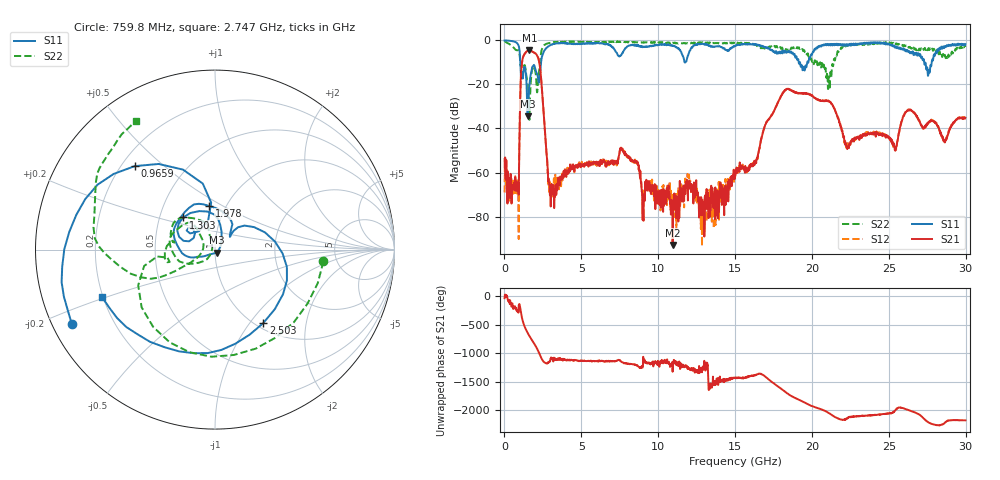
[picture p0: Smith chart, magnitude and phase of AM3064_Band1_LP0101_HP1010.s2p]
# Hz S DB R 50.0
!freq dBS11 angS11 dBS21 angS21 dBS12 angS12 dBS22 angS22
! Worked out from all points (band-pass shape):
!   1600 points, 10 MHz to 29.98 GHz, reference 50 ohm
!   highest |S21| = -4.58 dB at 1.622 GHz (marker M1); lowest = -92.9 dB at 10.94 GHz (marker M2)
!   |S21| within 3 dB of the highest: 1.212 GHz to 2.173 GHz (961.5 MHz wide, 56.8 % of centre)
!   lowest |S11| = -34.4 dB at 1.51 GHz (marker M3), VSWR 1.04, Z = 50.8 - j1.73 ohm
!   |S11| at or under -10 dB: 1.031 GHz to 2.382 GHz (1.351 GHz wide, 79.1 % of centre); 19.22 GHz to 19.69 GHz (470.1 MHz wide, 2.42 % of centre); 27.3 GHz to 27.79 GHz (490.7 MHz wide, 1.78 % of centre)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
!   |S22| runs from -36.1 to -0.4 dB; largest |S21 - S12| = 0.0095
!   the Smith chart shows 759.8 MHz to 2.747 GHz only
!   S11 on the Smith chart (normalised r, x): 759.8 MHz: 0.06, -0.24; 965.9 MHz: 0.25, +0.40; 1.303 GHz: 0.66, +0.25; 1.978 GHz: 0.83, +0.43; 2.503 GHz: 1.08, -1.17; 2.747 GHz: 0.20, -0.20
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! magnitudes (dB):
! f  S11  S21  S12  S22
! 10 MHz  0.0  -53.9  -69.1  -0.4
! 759.8 MHz  -0.9  -65.9  -64.4  -4.3
! 965.9 MHz  -3.8  -48.6  -48.9  -5.7
! 1.303 GHz  -12.0  -6.2  -6.2  -11.2
! 1.51 GHz  -34.4  -4.7  -4.7  -20.4
! 1.622 GHz  -20.4  -4.6  -4.5  -36.1
! 1.978 GHz  -12.2  -5.8  -5.7  -13.3
! 2.503 GHz  -6.2  -28.2  -28.1  -3.1
! 2.747 GHz  -3.3  -52.3  -51.5  -1.5
! 3.103 GHz  -2.0  -67.5  -70.9  -1.0
! 5.015 GHz  -1.5  -56.2  -57.1  -0.7
! 7.639 GHz  -6.0  -49.4  -49.4  -0.7
! 10 GHz  -2.0  -70.7  -74.1  -0.9
! 10.94 GHz  -2.3  -92.9  -71.2  -1.2
! 15 GHz  -2.6  -61.7  -61.8  -1.5
! 18.23 GHz  -5.4  -22.6  -22.8  -4.5
! 19.99 GHz  -6.6  -25.1  -25.1  -9.3
! 21.12 GHz  -1.8  -27.8  -27.6  -17.5
! 22.3 GHz  -2.3  -49.4  -48.2  -2.3
! 25 GHz  -1.5  -43.7  -44.5  -1.2
! 27.56 GHz  -15.9  -37.6  -37.6  -3.8
! 29.98 GHz  -1.7  -35.1  -35.4  -3.0
